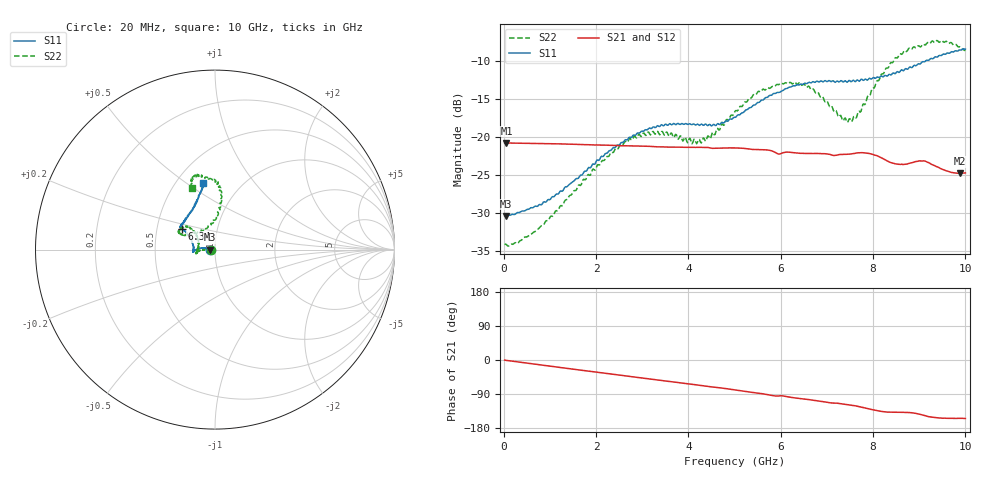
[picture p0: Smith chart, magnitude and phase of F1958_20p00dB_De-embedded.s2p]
! Integrated Device Technology
! Corporate Headquarters
! 6024 Silver Creek Valley Road
! San Jose, CA 95138  USA
! Phone:  1-408-284-8200
! Toll Free:  1-800-223-1366
! Webpage:  http://www.idt.com/
! Timing and RF Division
! 515 Groton Road, Suite 102
! Westford, MA 01886-6024
! Device:  F1958
! Description: 7-bit 0.25 dB Digital Step Attenuator
! Frequency:  0.001 -  6.000 GHz
! Package:  4x4 mm Thin QFN Plastic Package: 24 pin
! Ports:  2 RF, 12 DC
!  Pin  1  = D0
!  Pin  2  = VDD
!  Pin  3  = VMODE
!  Pin  4  = GND
!  Pin  5  = RF1  =  Port 1
!  Pin  6  = GND
!  Pin  7  = GND
!  Pin  8  = GND
!  Pin  9  = GND
!  Pin 10  = GND
!  Pin 11  = GND
!  Pin 12  = GND
!  Pin 13  = GND
!  Pin 14  = RF2  =  Port 2
!  Pin 15  = GND
!  Pin 16  = LE
!  Pin 17  = CLK
!  Pin 18  = DATA
!  Pin 19  = D6
!  Pin 20  = D5
!  Pin 21  = D4
!  Pin 22  = D3
!  Pin 23  = D2
!  Pin 24  = D1
! State:  80
! Atten State:  20.00 dB
! Voltage:  +3.30 Volts
! Current:  0.257 mA
! Data:  The device was measured on a F1958 evaluation board which has
!  individual transmission lines to the RF pins.  Data was collected
!  using a calibrated network analyzer.  The evaluation board was
!  de-embedded using Automatic Fixture Removal (AFR).
!  The reference plane is the edge of the package pin.
! Misc:
!  Action Tracker AT0419
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# GHz S dB R 50
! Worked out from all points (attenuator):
!   500 points, 20 MHz to 10 GHz, reference 50 ohm
!   highest |S21| = -20.78 dB at 60 MHz (marker M1); lowest = -24.8 dB at 9.88 GHz (marker M2)
!   lowest |S11| = -30.4 dB at 40 MHz (marker M3), VSWR 1.06, Z = 47.1 - j0.0427 ohm
!   |S11| at or under -10 dB: start of sweep to 9.142 GHz
!   |S22| runs from -34.3 to -7.3 dB; largest |S21 - S12| = 0.00038
!   S11 on the Smith chart (normalised r, x): 20 MHz: 0.94, -0.00; 6.34 GHz: 0.67, +0.16; 10 GHz: 0.67, +0.58
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0.02  -30.35 -178.9  -20.78 -0.4  -20.78 -0.4  -34.12 -177.8
0.04  -30.37 -179.1  -20.78 -0.7  -20.78 -0.7  -34.05 -177.1
0.06  -30.36 180.0  -20.78 -1.0  -20.78 -1.1  -34.12 -176.6
0.72  -29.11 172.9  -20.85 -11.7  -20.84 -11.6  -32.20 179.8
1.7  -24.96 171.6  -21.00 -27.1  -20.98 -27.1  -25.91 179.6
2.6  -20.62 177.5  -21.15 -41.2  -21.13 -41.2  -20.84 -175.8
3.36  -18.60 -175.1  -21.29 -53.2  -21.29 -53.3  -19.53 -167.8
4.26  -18.40 -179.4  -21.36 -67.0  -21.37 -67.0  -20.65 169.5
4.52  -18.47 174.6  -21.48 -71.3  -21.50 -71.3  -19.41 154.7
5.02  -17.41 161.4  -21.43 -79.1  -21.44 -79.1  -16.54 139.9
5.56  -15.29 150.8  -21.65 -88.3  -21.67 -88.3  -14.08 140.6
6.34  -13.18 148.0  -22.09 -100.6  -22.10 -100.5  -13.03 154.1
6.68  -12.79 146.8  -22.16 -105.6  -22.18 -105.5  -13.75 154.5
7.3  -12.60 141.1  -22.29 -115.3  -22.30 -115.2  -17.16 134.2
7.5  -12.62 138.4  -22.24 -118.6  -22.24 -118.5  -17.59 115.9
7.68  -12.58 135.5  -22.07 -122.4  -22.07 -122.4  -16.65 98.4
8.34  -11.80 119.4  -23.23 -137.7  -23.23 -137.8  -10.79 82.7
8.68  -11.17 112.6  -23.59 -138.3  -23.59 -138.1  -8.66 87.2
9.08  -10.10 107.4  -23.13 -145.4  -23.12 -145.4  -7.81 96.5
9.26  -9.68 104.9  -23.57 -150.5  -23.56 -150.6  -7.52 100.1
9.88  -8.56 100.3  -24.77 -154.0  -24.80 -154.0  -8.14 109.4
10  -8.47 99.9  -24.71 -154.3  -24.73 -154.4  -8.68 110.1
